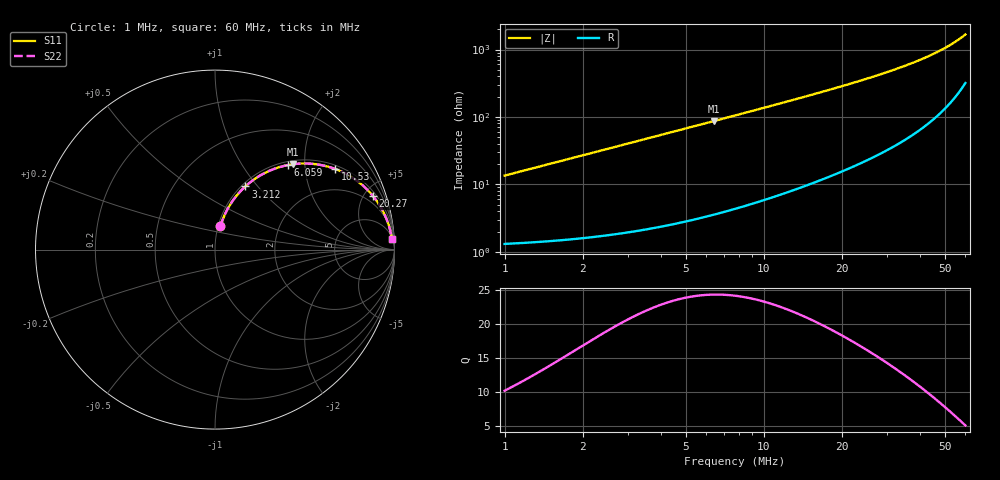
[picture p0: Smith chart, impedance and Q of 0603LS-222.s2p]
# MHz S MA R 50
!Freq  MagS11  AngS11  MagS21  AngS21  MagS12  AngS12  MagS22  AngS22
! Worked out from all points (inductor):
!   801 points, 1 MHz to 60 MHz, reference 50 ohm
!   read as one part in series: L = 2.14 uH near 1.021 MHz
!   highest Q = 24.4 at 6.41 MHz (marker M1), where L = 2.15 uH
!   S11 on the Smith chart (normalised r, x): 1 MHz: 1.03, +0.27; 3.212 MHz: 1.04, +0.86; 6.059 MHz: 1.07, +1.64; 10.53 MHz: 1.12, +2.87; 20.27 MHz: 1.32, +5.79; 60 MHz: 7, +33
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1  0.1322 76.9  0.9785 -7.6  0.9785 -7.6  0.1322 76.9
1.423526  0.186 75.1  0.9689 -10.7  0.9689 -10.7  0.186 75.1
1.915497  0.2463 72.3  0.9544 -14.2  0.9544 -14.2  0.2463 72.3
2.512373  0.3156 68.6  0.9326 -18.4  0.9326 -18.4  0.3156 68.6
3.211982  0.3906 64.4  0.9025 -23.0  0.9025 -23.0  0.3906 64.4
3.802961  0.4482 60.9  0.8743 -26.6  0.8743 -26.6  0.4482 60.9
4.479689  0.5077 57.1  0.8402 -30.5  0.8402 -30.5  0.5077 57.1
6.058799  0.6213 49.3  0.7585 -38.4  0.7585 -38.4  0.6213 49.3
6.409677  0.6422 47.7  0.7407 -39.9  0.7407 -39.9  0.6422 47.7
8.406954  0.7373 40.2  0.6456 -47.4  0.6456 -47.4  0.7373 40.2
10.53021  0.805 34.0  0.5595 -53.5  0.5595 -53.5  0.805 34.0
10.85858  0.8132 33.2  0.5476 -54.3  0.5476 -54.3  0.8132 33.2
12.79084  0.8531 28.9  0.4844 -58.5  0.4844 -58.5  0.8531 28.9
14.91351  0.8841 25.2  0.4269 -62.0  0.4269 -62.0  0.8841 25.2
17.38844  0.9095 21.8  0.3721 -65.3  0.3721 -65.3  0.9095 21.8
20.27408  0.9297 18.7  0.3209 -68.2  0.3209 -68.2  0.9297 18.7
20.6934  0.9321 18.3  0.3144 -68.5  0.3144 -68.5  0.9321 18.3
25.13588  0.9511 14.8  0.2558 -71.7  0.2558 -71.7  0.9511 14.8
30.53207  0.9648 11.7  0.2034 -74.2  0.2034 -74.2  0.9648 11.7
40.45798  0.9779 7.9  0.1373 -76.8  0.1373 -76.8  0.9779 7.9
50.41733  0.9841 5.2  0.09198 -77.4  0.09198 -77.4  0.9841 5.2
60  0.9871 3.3  0.05907 -75.7  0.05907 -75.7  0.9871 3.3
